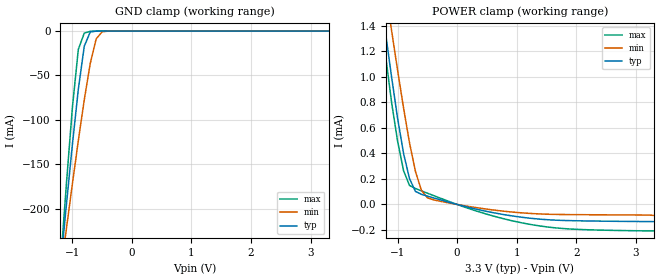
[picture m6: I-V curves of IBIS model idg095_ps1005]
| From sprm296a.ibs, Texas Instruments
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[Model]   idg095_ps1005
Model_type   Input
|  Input with 100 UA PULLUP
Polarity   Non-Inverting
| signals   A, Y
Vinl = 0.8V
Vinh = 2.0V
|   typ   min   max
C_comp   3.470p   3.429p   3.488p
|   typ   min   max
[Temperature Range]   25   -40   125
|   typ   min   max
[Voltage Range]   3.30V   3.00V   3.60V
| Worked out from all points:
|   GND clamp passes 1 mA (typ) near -0.70 V on its own axis
|   POWER clamp passes 1 mA (typ) near -1.10 V on its own axis
[GND_clamp]
|   Voltage   I(typ)   I(min)   I(max)
-3.3V     -1.82A     -1.4A      -2.328A
-1.2V     -265.4mA   -273.7mA   -263.5mA
-1.1V     -195.6mA   -222.6mA   -172.1mA
-1V       -128.1mA   -172.3mA   -86.5mA
-900mV    -65.59mA   -123.5mA   -20.61mA
-800mV    -17.01mA   -77.36mA   -2.282mA
-700mV    -1.036mA   -36.55mA   -230.6uA
-600mV    -43.17uA   -8.779mA   -13.26uA
-500mV    -2.108uA   -773.7uA   -463.6nA
-300mV    -3.791nA   -2.619uA   -288.7pA
3.3V      222pA      29.4nA     355.3pA
[POWER_clamp]
|   Voltage   I(typ)   I(min)   I(max)
-3.3V     9.016mA    8.661mA    9.714mA
-1.3V     1.684mA    1.994mA    1.543mA
-1.2V     1.335mA    1.674mA    1.159mA
-1.1V     995.1uA    1.359mA    796.1uA
-1V       674.2uA    1.051mA    495.5uA
-900mV    399.8uA    755.3uA    264.6uA
-800mV    201.5uA    482.5uA    148.7uA
-700mV    102.3uA    257.8uA    124.9uA
-600mV    79.32uA    110.4uA    106.6uA
-500mV    65.39uA    51.99uA    88.38uA
1.3V      -111.5uA   -72.32uA   -162.2uA
3.3V      -134.4uA   -85.62uA   -207.6uA
